DATA_BLOCK DB99
TITLE =

AUTHOR:INA
FAMILY:StateMac
NAME:nb
VERSION:00.00


    FB99


BEGIN
       Write:=FALSE
       NodeID:=B#16#00
       Mode:=B#16#00
       Done:=FALSE
       Err:=FALSE
       ErrNo:=L#0
       xEdgeMerker:=FALSE
       xEdgeFlag:=FALSE
       xStep:=0

END_DATA_BLOCK
